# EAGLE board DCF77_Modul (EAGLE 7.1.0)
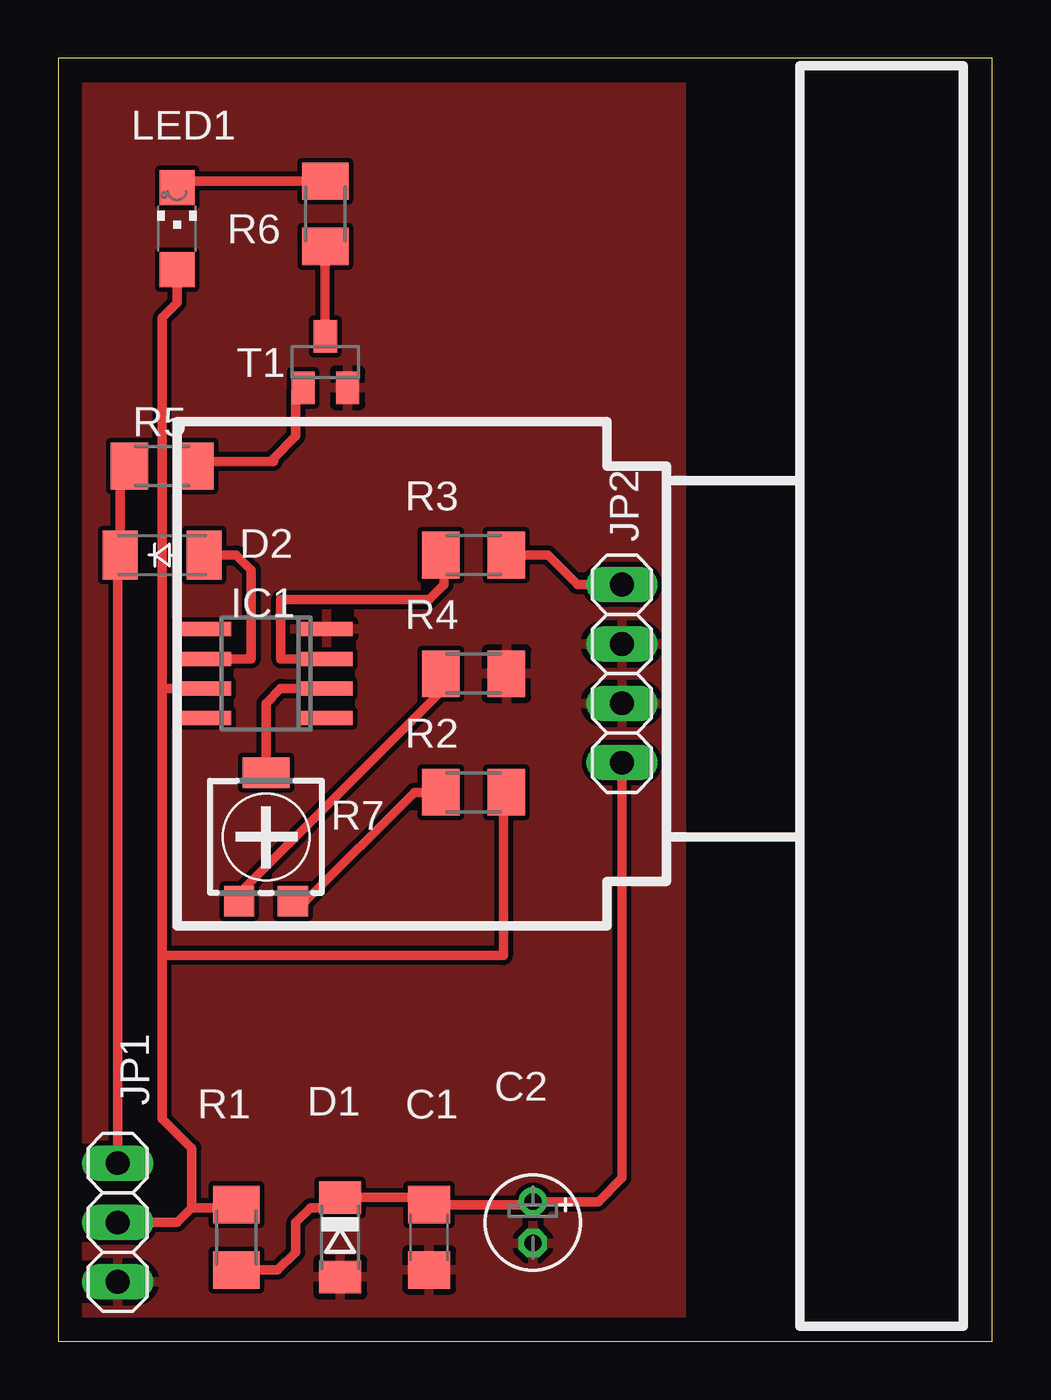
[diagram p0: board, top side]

Size 39.98 x 54.91 mm. Coordinates in mm from the lower left corner, seen from the top.
Outline: 0,0 39.98,0 39.98,54.91 0,54.91 0,0
Copper layers (1*16): Top 0.035mm / dielectric 1.5mm / Bottom 0.035mm
Design rules "default": minimum track width 10mil, minimum drill 24mil, track to track 8mil, track to pad 8mil, pad to pad 8mil, via to via 8mil, smd to smd 8mil, copper to edge 40mil, drill to drill 8mil, minimum pad ring 10mil, minimum via ring 8mil, stop-mask expansion 4mil, vias tented up to drill 0mil, thermal gap 10mil

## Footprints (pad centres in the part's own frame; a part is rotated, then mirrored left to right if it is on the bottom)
C1206 = smd 1.6 x 1.8: 1 -1.4,0; 2 1.4,0
E1,8-4 = drill 0.711 pad 1.168: + -0.889,0 | drill 0.711 pad 1.168 octagon: - 0.889,0
SOD80C = smd 1.4 x 1.8: A 1.7,0; C -1.7,0
SOD-123_MINI-SMA = smd 1.5 x 2.1: A 1.8,0; C -1.8,0
SO08 = smd 0.6 x 2.2: 1 -1.905,-2.6; 2 -0.635,-2.6; 3 0.635,-2.6; 4 1.905,-2.6; 5 1.905,2.6; 6 0.635,2.6; 7 -0.635,2.6; 8 -1.905,2.6
1X03 = drill 1.016 long: 1 -2.54,0; 2 0,0; 3 2.54,0
1X04 = drill 1.016 long: 1 -3.81,0; 2 -1.27,0; 3 1.27,0; 4 3.81,0
CHIPLED_1206 = smd 1.5 x 1.5: A 0,-1.75; C 0,1.75
M1206 = smd 1.6 x 2: 1 -1.4,0; 2 1.4,0
RTRIM4G/J = smd 1.3 x 1.3: 1 -1.15,-2.75; 3 1.15,-2.75 | smd 2 x 1.3: 2 0,2.75
SOT23 = smd 1 x 1.4: 1 -0.95,-1.1; 2 0.95,-1.1; 3 0,1.1

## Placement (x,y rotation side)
C1  100n  [C1206]  15.88,4.45 270 top
C2  10u  [E1,8-4]  20.32,5.08 270 top
D1  3,9  [SOD80C]  12.06,4.45 270 top
D2  [SOD-123_MINI-SMA]  4.45,33.66 0 top
IC1  TL061D  [SO08]  8.89,28.57 90 top
JP1  RasPi  [1X03]  2.54,5.08 90 top
JP2  DCF77-Modul  [1X04]  24.13,28.57 90 top
LED1  [CHIPLED_1206]  5.08,47.62 0 top
R1  680  [M1206]  7.62,4.45 270 top
R2  100k  [M1206]  17.78,23.5 0 top
R3  100k  [M1206]  17.78,33.66 180 top
R4  100k  [M1206]  17.78,28.57 180 top
R5  47k  [M1206]  4.45,37.47 0 top
R6  1k  [M1206]  11.43,48.26 90 top
R7  100k  [RTRIM4G/J]  8.89,21.59 0 top
T1  BC847  [SOT23]  11.43,41.91 0 top

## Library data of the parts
C1 C2 R1-R7 = rcl
D1 D2 = diode
IC1 = linear
JP1 JP2 = pinhead
LED1 = led
T1 = transistor

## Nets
3,9V: C1.1 C2.+ D1.C JP2.1 R1.2
DCF: JP2.4 R3.1
DIGITALOUT: D2.C JP1.3 R5.1
GND: C1.2 C2.- D1.A IC1.4 JP1.1 JP2.2 JP2.3 R4.1 T1.2
N$5: R4.2 R7.1
N$6: R2.1 R7.3
N$7: IC1.2 R7.2
N$8: IC1.3 R3.2
N$11: D2.A IC1.6
N$12: R5.2 T1.1
N$13: R6.1 T1.3
N$14: LED1.C R6.2
VCC: IC1.7 JP1.2 LED1.A R1.1 R2.2

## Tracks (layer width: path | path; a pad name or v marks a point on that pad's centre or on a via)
3,9V
  Top 0.406: R1.2 9.39,3.04 10.16,3.81 10.16,5.08 10.79,5.71 11.63,5.71 D1.C 15.57,6.14 C1.1 19.81,5.84 C2.+ 23.11,5.97 24.13,6.99 JP2.1
DCF
  Top 0.406: JP2.4 22.23,32.38 20.95,33.66 R3.1
DIGITALOUT
  Top 0.406: R5.1 2.65,37.06 D2.C 2.65,33.12 2.54,33.02 JP1.3
GND
  Top 0.406: 15.88,2.54 C1.2
  pour Top: 0.64,53.98 26.67,53.98 26.67,0.64 0.64,0.64
N$5
  Top 0.406: R7.1 7.74,19.17 16.51,27.94 16.51,28.45 R4.2
N$6
  Top 0.406: R7.3 10.59,18.84 15.24,23.5 R2.1
N$7
  Top 0.406: R7.2 8.89,27.3 9.53,27.94 IC1.2
N$8
  Top 0.406: IC1.3 9.53,29.21 9.53,31.75 15.88,31.75 16.51,32.38 16.51,33.52 R3.2
N$11
  Top 0.406: D2.A 7.62,33.66 8.26,33.02 8.26,29.21 IC1.6
N$12
  Top 0.406: T1.1 10.16,40.64 10.16,38.73 9.21,37.78 9.21,37.66 6.04,37.66 R5.2
N$13
  Top 0.406: T1.3 R6.1
N$14
  Top 0.406: R6.2 5.08,49.66 LED1.C
VCC
  Top 0.406: JP1.2 5.08,5.08 5.71,5.71 | 6.99,5.71 7.49,5.71 R1.1 7.62,6.35 6.99,5.71 | 19.05,22.86 19.05,23.36 R2.2 19.18,22.99 19.05,22.86 | 19.05,22.86 19.05,16.51 4.45,16.51 | 4.45,16.51 4.45,27.94 | IC1.7 4.45,27.94 | 4.45,27.94 4.45,43.81 5.08,44.45 LED1.A | 6.99,5.71 5.71,5.71 | 5.71,5.71 5.71,8.26 4.45,9.53 4.45,16.51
